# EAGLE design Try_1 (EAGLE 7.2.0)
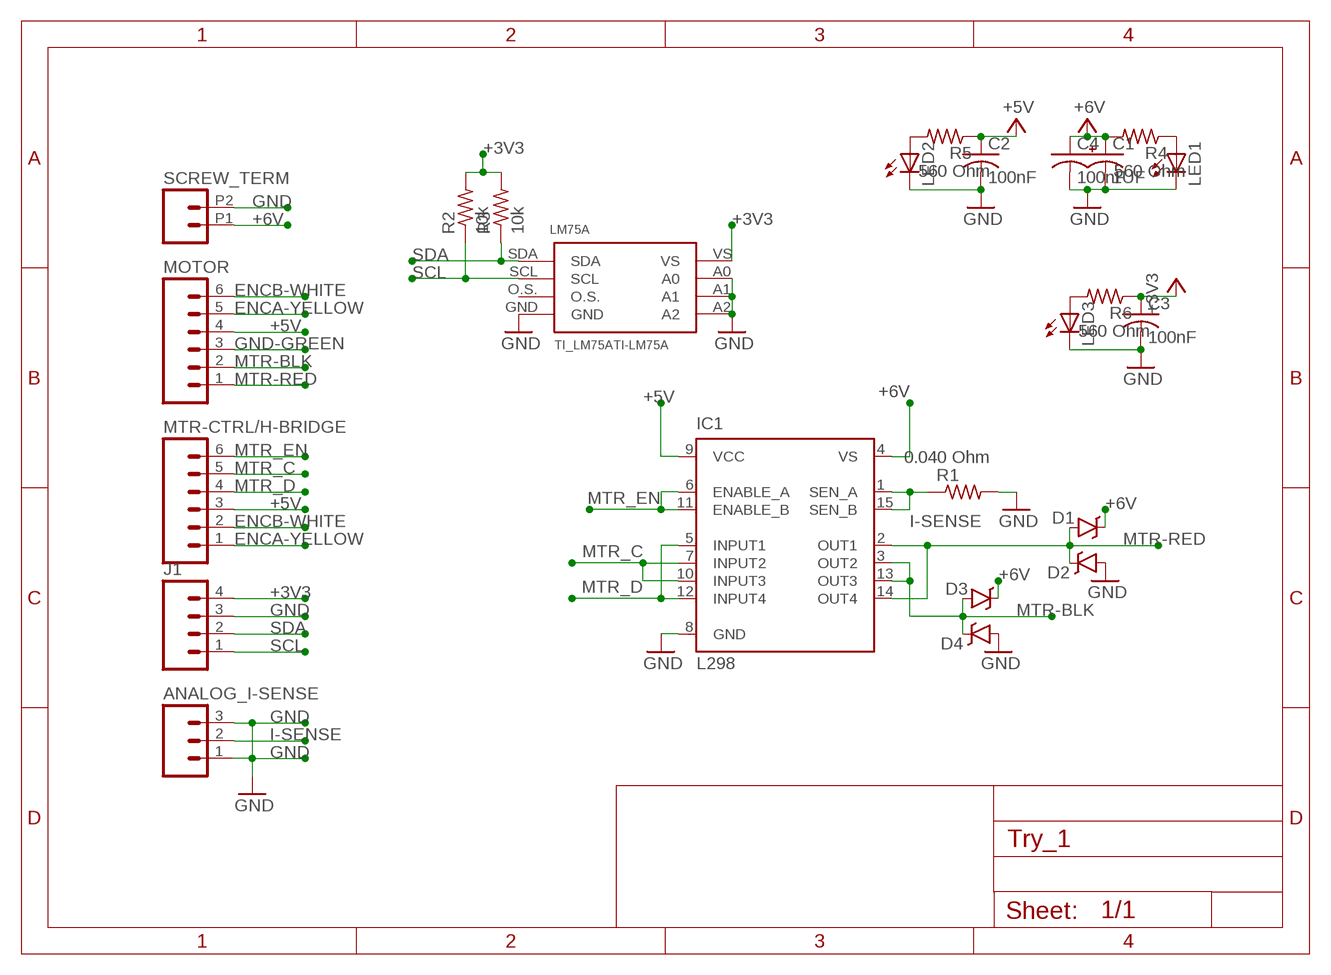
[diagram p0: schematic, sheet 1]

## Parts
ANALOG_I-SENSE  M03PTH  [1X03]
C1  1UF  1UF-50V-20%(PTH)KIT  [CPOL-RADIAL-1UF-50V-KIT]
C2  100nF  C-USC1206  [C1206]
C3  100nF  C-USC1206  [C1206]
C4  100nF  C-USC1206  [C1206]
D1  B340A  DIODE-SCHOTTKY-B340A  [SMA-DIODE]
D2  B340A  DIODE-SCHOTTKY-B340A  [SMA-DIODE]
D3  B340A  DIODE-SCHOTTKY-B340A  [SMA-DIODE]
D4  B340A  DIODE-SCHOTTKY-B340A  [SMA-DIODE]
IC1  L298  [MULTIWATT-15]
J1  M04PTH  [1X04]
LED1  LEDSMT1206  [1206]
LED2  LEDSMT1206  [1206]
LED3  LEDSMT1206  [1206]
LM75A  TI_LM75ATI-LM75A  [TI_LM75A]
MOTOR  M06SILK_FEMALE_PTH  [1X06]
MTR-CTRL/H-BRIDGE  M06SILK_FEMALE_PTH  [1X06]
R1  0.040 Ohm  R-US_M1206  [M1206]
R2  10k  R-US_M1206  [M1206]
R3  10k  R-US_M1206  [M1206]
R4  560 Ohm  R-US_M1206  [M1206]
R5  560 Ohm  R-US_M1206  [M1206]
R6  560 Ohm  R-US_M1206  [M1206]
SCREW_TERM  M022.54MM_SCREWTERM  [1X02_2.54_SCREWTERM]

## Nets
+3V3: C3.1 J1.4 LM75A.VS R2.2 R3.2 R6.1
+5V: C2.1 IC1.9(VCC) MOTOR.4 MTR-CTRL/H-BRIDGE.3 R5.1
+6V: C1.1(+) C4.1 D1.C D3.C IC1.4(VS) R4.2 SCREW_TERM.P1
ENCA-YELLOW: MOTOR.5 MTR-CTRL/H-BRIDGE.1
ENCB-WHITE: MOTOR.6 MTR-CTRL/H-BRIDGE.2
GND: ANALOG_I-SENSE.1 ANALOG_I-SENSE.3 C1.2(-) C2.2 C3.2 C4.2 D2.A D4.A IC1.8(GND) J1.3 LED1.C LED2.C LED3.C LM75A.A0 LM75A.A1 LM75A.A2 LM75A.GND R1.2 SCREW_TERM.P2
GND-GREEN: MOTOR.3
I-SENSE: ANALOG_I-SENSE.2 IC1.1(SEN_A) IC1.15(SEN_B) R1.1
MTR-BLK: D3.A D4.C IC1.3(OUT2) IC1.13(OUT3) MOTOR.2
MTR-RED: D1.A D2.C IC1.2(OUT1) IC1.14(OUT4) MOTOR.1
MTR_C: IC1.7(INPUT2) IC1.10(INPUT3) MTR-CTRL/H-BRIDGE.5
MTR_D: IC1.5(INPUT1) IC1.12(INPUT4) MTR-CTRL/H-BRIDGE.4
MTR_EN: IC1.6(ENABLE_A) IC1.11(ENABLE_B) MTR-CTRL/H-BRIDGE.6
N$2: LED1.A R4.1
N$3: LED2.A R5.2
N$4: LED3.A R6.2
SCL: J1.1 LM75A.SCL R2.1
SDA: J1.2 LM75A.SDA R3.1
Unconnected: LM75A.O.S.

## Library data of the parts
ANALOG_I-SENSE = SparkFun-Connectors:M03: Header 3 Standard 3-pin 0.1" header. Use with straight break away headers (SKU : PRT-00116), right angle break away headers (PRT-00553), swiss pins (PRT-00743), machine pins (PRT-00117), and female headers (PRT-00115). Molex polarized connector foot print use with SKU : PRT-08232 with associated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
C1 = MORE_CAPS:1UF-50V-20%(PTH): CAP ALUM 1UF 20% 50V RADIAL; PROD_ID: USR1H010MDD
C2-C4 = rcl:C-US: CAPACITOR, American symbol
D1-D4 = SparkFun-DiscreteSemi:DIODE-SCHOTTKY: Schottky diodes in SFE's production catalog; PROD_ID: DIO-09886
IC1 = st-microelectronics:L298: DUAL FULL-BRIDGE DRIVER; MPN: L298N; OC_FARNELL: 1589425; OC_NEWARK: 32M1527
J1 = SparkFun-Connectors:M04: Header 4 Standard 4-pin 0.1" header. Use with straight break away headers (SKU : PRT-00116), right angle break away headers (PRT-00553), swiss pins (PRT-00743), machine pins (PRT-00117), and female headers (PRT-00115). Molex polarized connector foot print use with SKU : PRT-08231 with associated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; PROD_ID: CONN-09696
LED1-LED3 = led:LED: LED
LM75A = TI-LM75A:TI_LM75A: 8pin SPI Flash series x25xx. Works with devices like W25X32 and BR25L32
MOTOR MTR-CTRL/H-BRIDGE = SparkFun-Connectors:M06: Header 6 Standard 6-pin 0.1" header. Use with straight break away headers (SKU : PRT-00116), right angle break away headers (PRT-00553), swiss pins (PRT-00743), machine pins (PRT-00117), and female headers (PRT-00115). Molex polarized connector foot print use with SKU : PRT-08094 with associated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; PROD_ID: CONN-08437
R1-R6 = rcl:R-US_: RESISTOR, American symbol
SCREW_TERM = SparkFun-Connectors:M02: Standard 2-pin 0.1" header. Use with

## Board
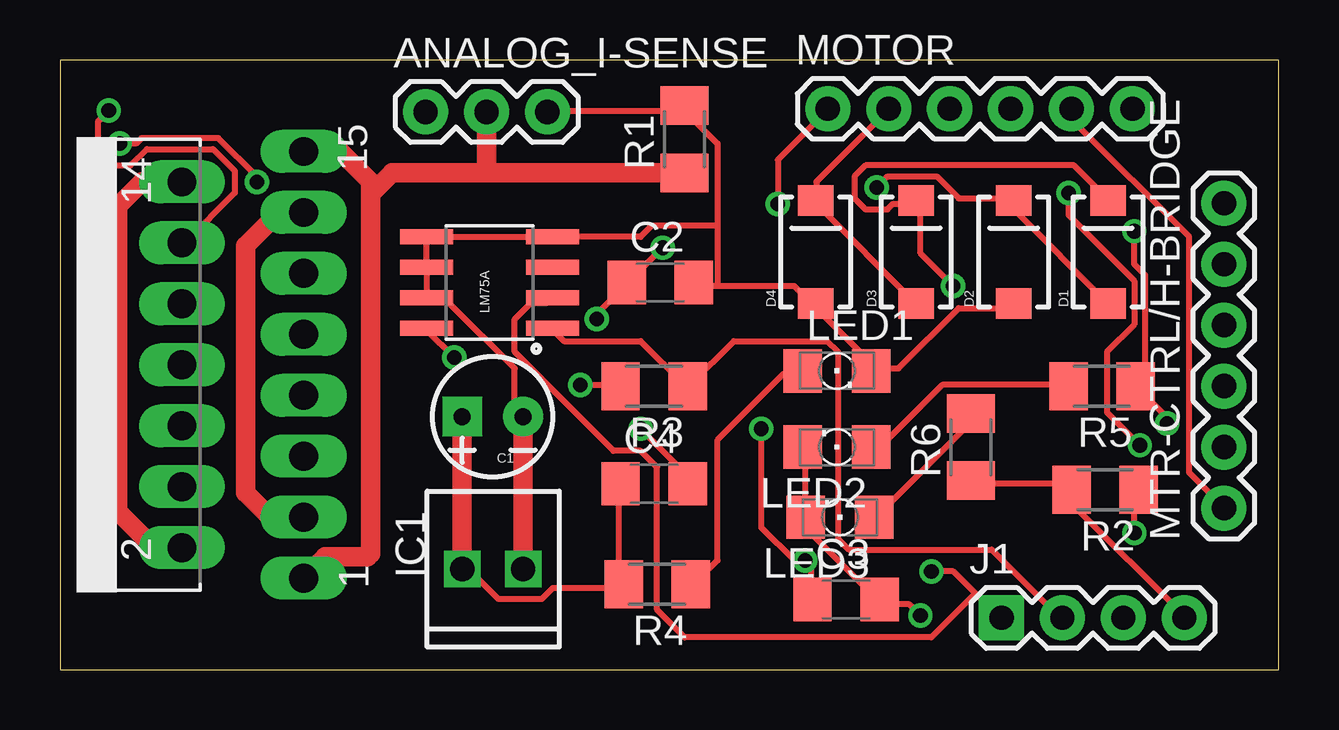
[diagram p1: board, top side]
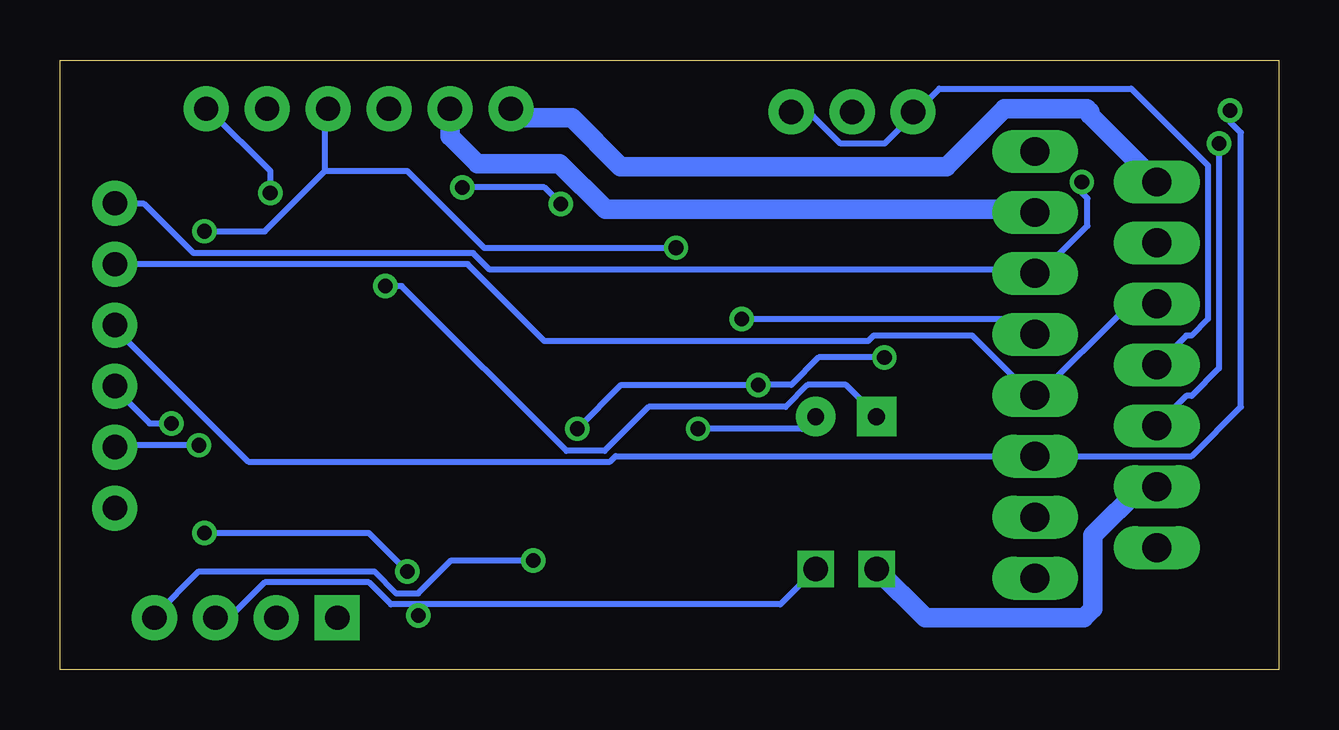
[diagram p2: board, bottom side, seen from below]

Size 50.8 x 25.4 mm. Coordinates in mm from the lower left corner, seen from the top.
Outline: 0,0 50.8,0 50.8,25.4 0,25.4 0,0
Copper layers (1*16): Top 0.035mm / dielectric 1.5mm / Bottom 0.035mm
Design rules "default": minimum track width 10mil, minimum drill 24mil, track to track 8mil, track to pad 8mil, pad to pad 8mil, via to via 8mil, smd to smd 8mil, copper to edge 40mil, drill to drill 8mil, minimum pad ring 10mil, minimum via ring 8mil, stop-mask expansion 4mil, vias tented up to drill 0mil, thermal gap 10mil

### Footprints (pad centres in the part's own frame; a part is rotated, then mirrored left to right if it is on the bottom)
1X03 = drill 1.016 pad 1.88: 1 0,0; 2 2.54,0; 3 5.08,0
CPOL-RADIAL-1UF-50V-KIT = drill 0.7 pad 1.651 square: 1 1.27,0 | drill 0.7 pad 1.651: 2 -1.27,0
C1206 = smd 1.6 x 1.8: 1 -1.4,0; 2 1.4,0
SMA-DIODE = smd 1.27 x 1.47: A -2.15,0; C 2.15,0
MULTIWATT-15 = drill 1.2 long: 1 -8.89,-7.62; 2 -7.62,-2.54; 3 -6.35,-7.62; 4 -5.08,-2.54; 5 -3.81,-7.62; 6 -2.54,-2.54; 7 -1.27,-7.62; 8 0,-2.54; 9 1.27,-7.62; 10 2.54,-2.54; 11 3.81,-7.62; 12 5.08,-2.54; 13 6.35,-7.62; 14 7.62,-2.54; 15 8.89,-7.62
1X04 = drill 1.016 pad 1.88 square: 1 0,0 | drill 1.016 pad 1.88: 2 2.54,0; 3 5.08,0; 4 7.62,0
1206 = smd 1.6 x 1.803: A -1.422,0; C 1.422,0
TI_LM75A = smd 0.61 x 2.21: A0 -0.635,2.616; A1 0.635,2.616; A2 1.905,2.616; GND 1.905,-2.616; O.S. 0.635,-2.616; SCL -0.635,-2.616; SDA -1.905,-2.616; VS -1.905,2.616
1X06 = drill 1.016 pad 1.88: 1 0,0; 2 2.54,0; 3 5.08,0; 4 7.62,0; 5 10.16,0; 6 12.7,0
M1206 = smd 1.6 x 2: 1 -1.4,0; 2 1.4,0
1X02_2.54_SCREWTERM = drill 1.016 square: P1 2.54,0; P2 0,0

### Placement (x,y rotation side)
ANALOG_I-SENSE  15.24,23.24 0 top
C1  18.03,10.54 180 top
C2  25.02,16.13 0 top
C3  32.77,2.92 0 top
C4  24.77,7.75 0 top
D1  43.69,17.4 90 top
D2  39.75,17.4 90 top
D3  35.69,17.4 90 top
D4  31.5,17.4 90 top
IC1  2.54,12.7 90 top
J1  39.24,2.16 0 top
LED1  32.39,12.45 0 top
LED2  32.39,9.27 180 top
LED3  32.51,6.35 180 top
LM75A  17.91,16.13 90 top
MOTOR  32,23.37 0 top
MTR-CTRL/H-BRIDGE  48.51,6.73 90 top
R1  26.04,22.1 90 top
R2  43.56,7.49 180 top
R3  24.77,11.81 180 top
R4  24.89,3.56 180 top
R5  43.43,11.81 180 top
R6  37.97,9.27 90 top
SCREW_TERM  19.3,4.19 180 top

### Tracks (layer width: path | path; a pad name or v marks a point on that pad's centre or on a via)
+3V3  (via drill 0.61)
  Top 0.254: v21.69,11.86 23.29,11.86 R3.2 | v16.43,13 15.29,14.15 LM75A.VS | R6.1 38.15,7.75 41.81,7.75 42.04,7.52 R2.2 42.27,7.29 42.27,6.83 46.84,2.26 J1.4 | C3.1 31.29,2.95 31.29,4.32 v31.06,4.55 30.61,4.55 29.23,5.92 v29.23,10.03
  Bottom 0.254: v16.43,13 19.18,13 20.32,11.86 v21.69,11.86 27.41,11.86 v29.23,10.03 | v31.06,4.55 34.49,4.55 35.87,3.17 36.78,3.17 37.69,4.09 45.01,4.09 46.84,2.26 J1.4
+5V  (via drill 0.61)
  Top 0.254: v22.38,14.61 22.38,14.83 23.52,15.98 C2.1 23.75,16.2 v25.12,17.58 | v46.15,10.26 46.15,10.49 45.01,11.63 R5.1 45.01,11.86 45.24,12.09 45.24,16.43 44.78,16.89 v44.78,18.26
  Bottom 0.254: v22.38,14.61 10.72,14.61 10.26,14.15 IC1.9 | v46.15,10.26 47.07,10.26 48.44,11.63 MTR-CTRL/H-BRIDGE.3 | 39.75,20.78 39.75,23.29 MOTOR.4 | 39.75,20.78 42.27,18.26 v44.78,18.26 | v25.12,17.58 33.12,17.58 36.32,20.78 39.75,20.78
+6V  (via drill 0.61)
  Top 0.254: D1.C 43.64,19.63 42.27,21.01 33.58,21.01 33.12,20.55 33.12,19.63 33.58,19.18 34.49,19.18 34.72,19.41 35.64,19.41 D3.C 35.87,19.41 35.87,17.35 v37.24,15.98 | C4.1 23.29,7.75 23.29,3.63 R4.2 23.29,3.4 20.55,3.4 20.09,2.95 18.26,2.95 17.12,4.09 SCREW_TERM.P1
  Top 0.813: SCREW_TERM.P1 C1.1
  Bottom 0.254: v37.24,15.98 36.55,15.98 29.69,9.12 28.09,9.12 26.26,10.95 20.55,10.95 19.63,11.86 18.03,11.86 16.89,10.72 C1.1
  Bottom 0.813: IC1.4 5.72,7.62 7.75,5.59 7.75,2.54 8.13,2.16 14.73,2.16 SCREW_TERM.P1
ENCA-YELLOW
  Top 0.254: MOTOR.5 42.27,23.29 42.27,22.84 47.07,18.03 47.07,8.2 48.44,6.83 MTR-CTRL/H-BRIDGE.1
ENCB-WHITE  (via drill 0.61)
  Top 0.254: v45.01,9.35 43.64,10.72 43.64,13.23 44.78,14.38 44.78,16.2 42.04,18.95 v42.04,19.86
  Bottom 0.254: v45.01,9.35 48.44,9.35 MTR-CTRL/H-BRIDGE.2 | v42.04,19.86 42.04,20.78 44.55,23.29 MOTOR.6
GND  (via drill 0.61)
  Top 0.254: LED2.C 31.06,9.12 31.06,6.38 LED3.C 31.29,6.15 31.29,5.69 34.04,2.95 C3.2 34.27,2.72 35.41,2.72 v35.87,2.26 | v24.21,10.03 26.04,8.2 26.04,7.75 C4.2 | C1.2 18.95,10.72 18.95,12.55 16.21,15.29 15.29,15.29 LM75A.A0 LM75A.A1 LM75A.A2 LM75A.GND 24.21,18.03 24.66,18.49 27.41,18.49 | D2.A 39.75,15.06 37.47,15.06 34.95,12.55 33.81,12.55 LED1.C 33.58,12.55 33.58,13 31.52,15.06 D4.A 31.29,15.29 30.61,15.98 27.41,15.98 | 27.41,15.98 26.49,15.98 C2.2 | 26.04,23.29 20.32,23.29 ANALOG_I-SENSE.3 | 27.41,18.49 27.41,21.92 26.04,23.29 | 27.41,18.49 27.41,15.98 | 26.04,23.29 R1.2
  Top 0.813: SCREW_TERM.P2 C1.2
  Bottom 0.254: v24.21,10.03 19.86,10.03 19.41,10.49 C1.2 | 35.87,2.72 20.78,2.72 SCREW_TERM.P2 | 35.87,2.72 37.01,2.72 37.92,3.63 42.27,3.63 43.64,2.26 44.32,2.26 J1.3 | 35.87,2.72 v35.87,2.26 | IC1.8 3.86,13.92 3.63,13.92 2.95,14.61 2.95,21.01 6.15,24.21 14.15,24.21 15.06,23.29 ANALOG_I-SENSE.1 15.29,23.06 16.43,21.92 18.26,21.92 19.41,23.06 20.32,23.06 ANALOG_I-SENSE.3
I-SENSE
  Top 0.813: IC1.15 11.68,21.59 12.95,20.32 12.95,19.81 | 12.95,19.81 12.95,4.83 12.83,4.7 11.05,4.7 IC1.1 | R1.1 18.03,20.7 | 18.03,20.7 13.84,20.7 12.95,19.81 | ANALOG_I-SENSE.2 17.78,20.95 18.03,20.7
MTR-BLK
  Top 0.254: D3.A 35.64,15.29 31.52,19.41 D4.C 31.52,19.63 31.52,20.32 34.49,23.29 MOTOR.2
  Top 0.813: IC1.3 8.76,6.35 7.75,7.37 7.75,17.65 9.14,19.05 IC1.13
  Bottom 0.813: IC1.13 10.29,19.18 28.07,19.18 29.97,21.08 33.4,21.08 34.54,22.22 MOTOR.2
MTR-RED  (via drill 0.61)
  Top 0.254: D1.A 43.64,15.29 39.75,19.18 D2.C 39.75,19.63 37.47,19.63 36.55,20.55 34.49,20.55 v34.04,20.09 | v29.92,19.41 29.92,21.23 31.98,23.29 MOTOR.1
  Top 0.813: IC1.14 3.43,20.32 2.41,19.3 2.41,6.6 3.81,5.21 4.95,5.21 IC1.2
  Bottom 0.254: v34.04,20.09 30.61,20.09 v29.92,19.41
  Bottom 0.813: IC1.14 7.87,23.11 7.87,23.24 8,23.37 11.43,23.37 13.84,20.95 27.43,20.95 29.46,22.99 31.62,22.99 MOTOR.1
MTR_C
  Bottom 0.254: IC1.10 5.23,15.06 6.38,15.06 10.03,11.41 IC1.7 10.26,11.41 12.78,13.92 16.89,13.92 17.12,13.69 30.61,13.69 33.81,16.89 MTR-CTRL/H-BRIDGE.5
MTR_D  (via drill 0.61)
  Top 0.254: v2.03,23.29 1.58,22.84 1.58,21.46 2.03,21.01 2.95,21.01 3.63,21.69 6.38,21.69 7.29,20.78 7.29,19.86 5.23,17.8 IC1.12
  Bottom 0.254: MTR-CTRL/H-BRIDGE.4 48.44,14.15 42.95,8.66 27.86,8.66 27.64,8.89 IC1.5 3.63,8.89 1.58,10.95 1.58,22.38 2.03,22.84 v2.03,23.29
MTR_EN  (via drill 0.61)
  Top 0.254: v2.49,21.92 3.18,21.92 3.4,22.15 6.6,22.15 8.2,20.55 v8.2,20.32
  Bottom 0.254: v2.49,21.92 2.49,12.55 3.63,11.41 3.86,11.41 5,10.26 IC1.6 | v8.2,20.32 8.2,19.86 7.98,19.63 7.98,18.49 10.03,16.43 IC1.11 10.26,16.66 32.89,16.66 33.58,17.35 45.24,17.35 47.3,19.41 48.44,19.41 MTR-CTRL/H-BRIDGE.6
N$2
  Top 0.254: LED1.A 30.84,12.32 30.15,12.32 27.41,9.58 27.41,4.55 26.49,3.63 R4.1
N$3
  Top 0.254: LED2.A 33.81,9.35 34.27,9.35 36.78,11.86 41.81,11.86 R5.2
N$4
  Top 0.254: LED3.A 34.04,6.38 38.15,10.49 R6.2
SCL  (via drill 0.61)
  Top 0.254: v44.78,5.69 44.78,7.29 R2.1 | v36.32,4.09 37.24,4.09 38.15,3.17 | 38.15,3.17 39.06,2.26 J1.1 | 38.15,3.17 36.32,1.35 26.04,1.35 24.89,2.49 24.89,8.43 24.21,9.12 23.06,9.12 18.95,13.23 18.95,14.61 19.63,15.29 20.32,15.29 LM75A.SCL
  Bottom 0.254: v44.78,5.69 37.92,5.69 v36.32,4.09
SDA
  Top 0.254: LM75A.SDA 20.55,14.15 21.01,13.69 24.21,13.69 26.04,11.86 R3.1 26.26,11.86 28.09,13.69 31.98,13.69 32.44,13.23 32.44,5.46 32.89,5 38.84,5 41.58,2.26 J1.2

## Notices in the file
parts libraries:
SparkFun-Connectors: Licensing: Creative Commons ShareAlike 4.0 International - https://creativecommons.org/licenses/by-sa/4.0
